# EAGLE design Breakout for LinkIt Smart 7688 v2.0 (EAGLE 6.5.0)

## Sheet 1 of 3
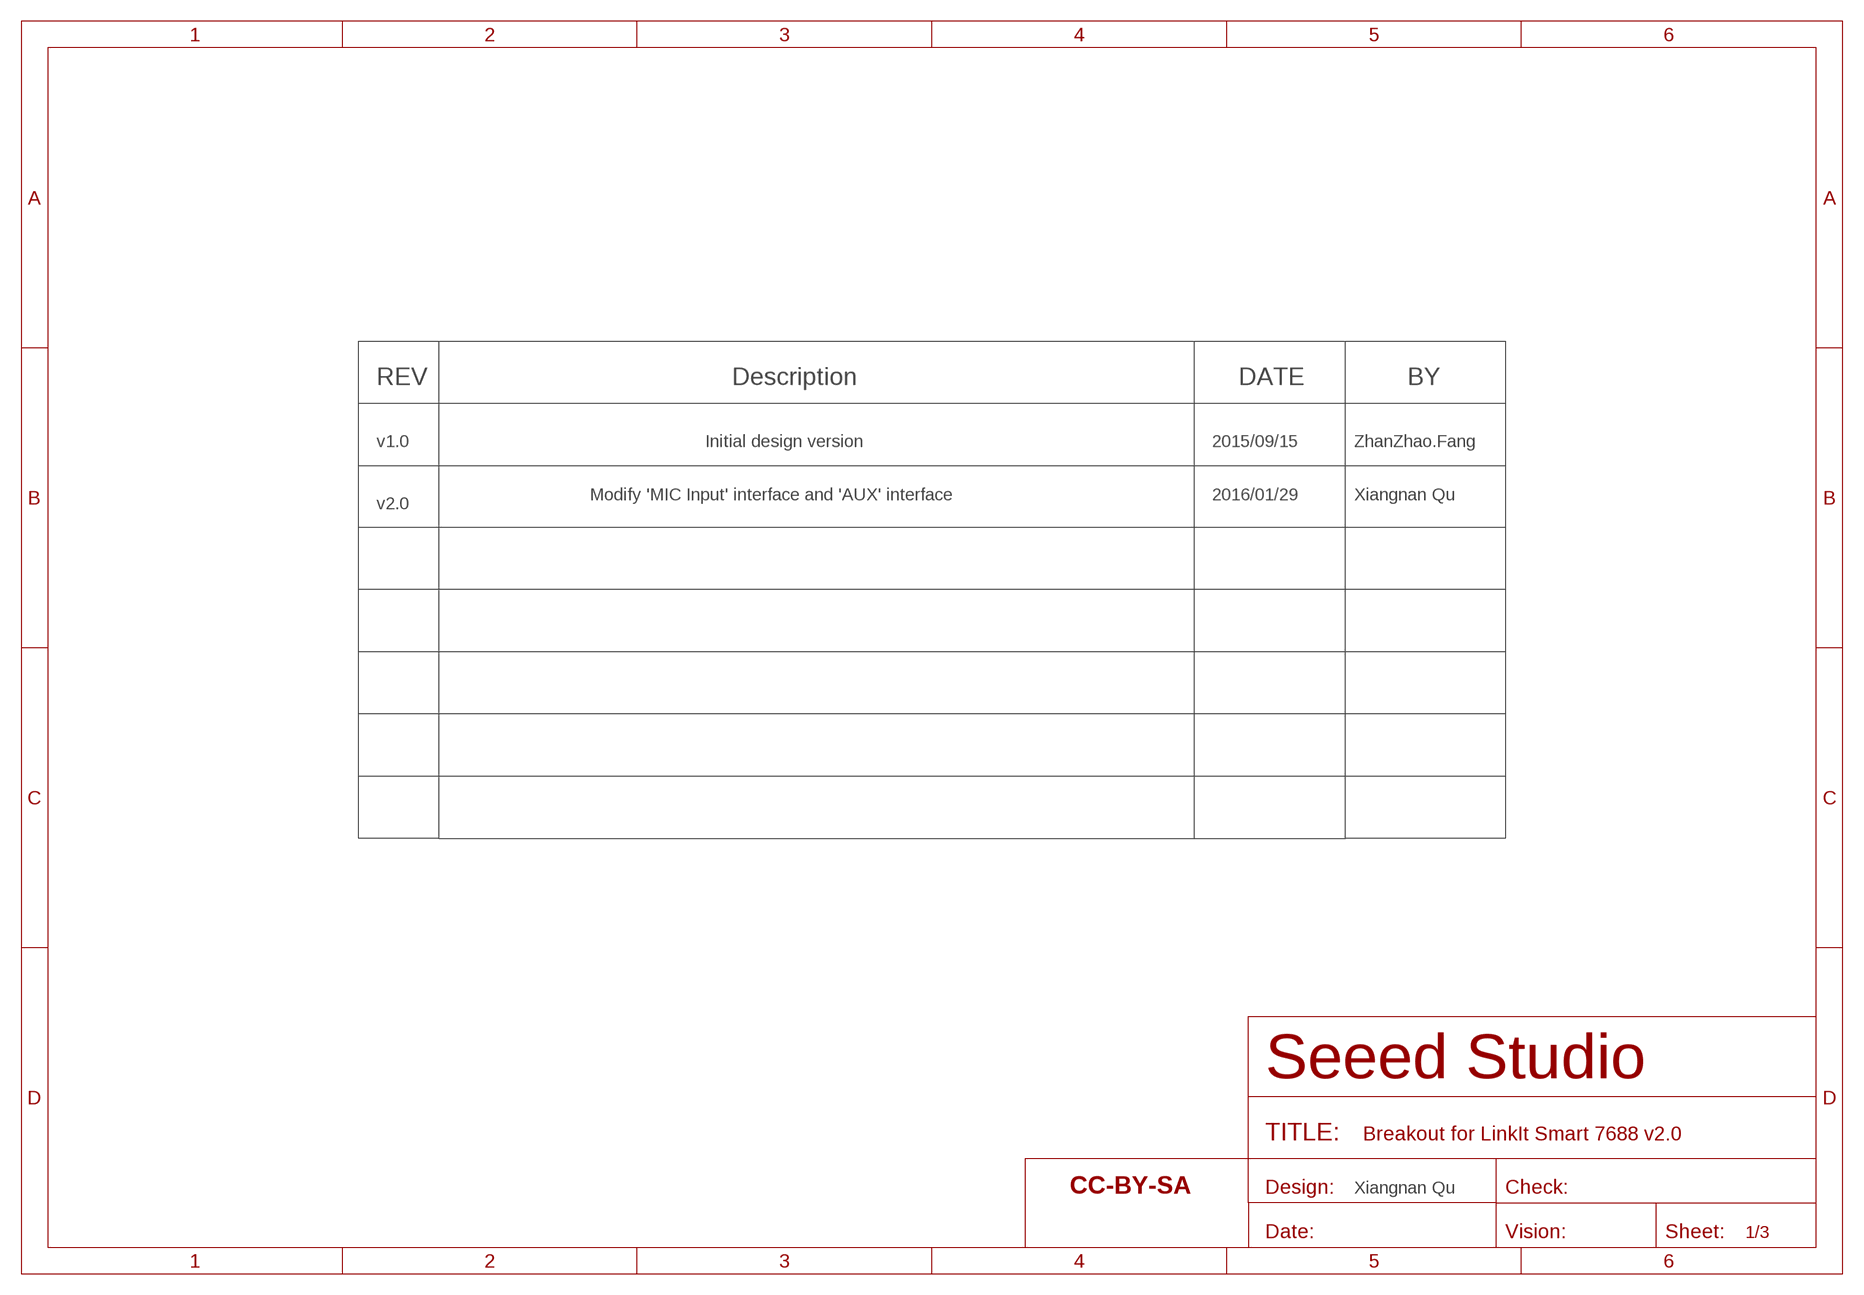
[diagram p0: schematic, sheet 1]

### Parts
FR2  DNP  SEEEDSTUDIO-OPEN-SCH-FRAME  [SEEEDSTUDIO-PCB-FRAME]

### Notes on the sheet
- REV | Description | DATE | BY
- v1.0 | Initial design version | 2015/09/15 | ZhanZhao.Fang
- Modify 'MIC Input' interface and 'AUX' interface | 2016/01/29 | Xiangnan Qu
- v2.0
- Xiangnan Qu

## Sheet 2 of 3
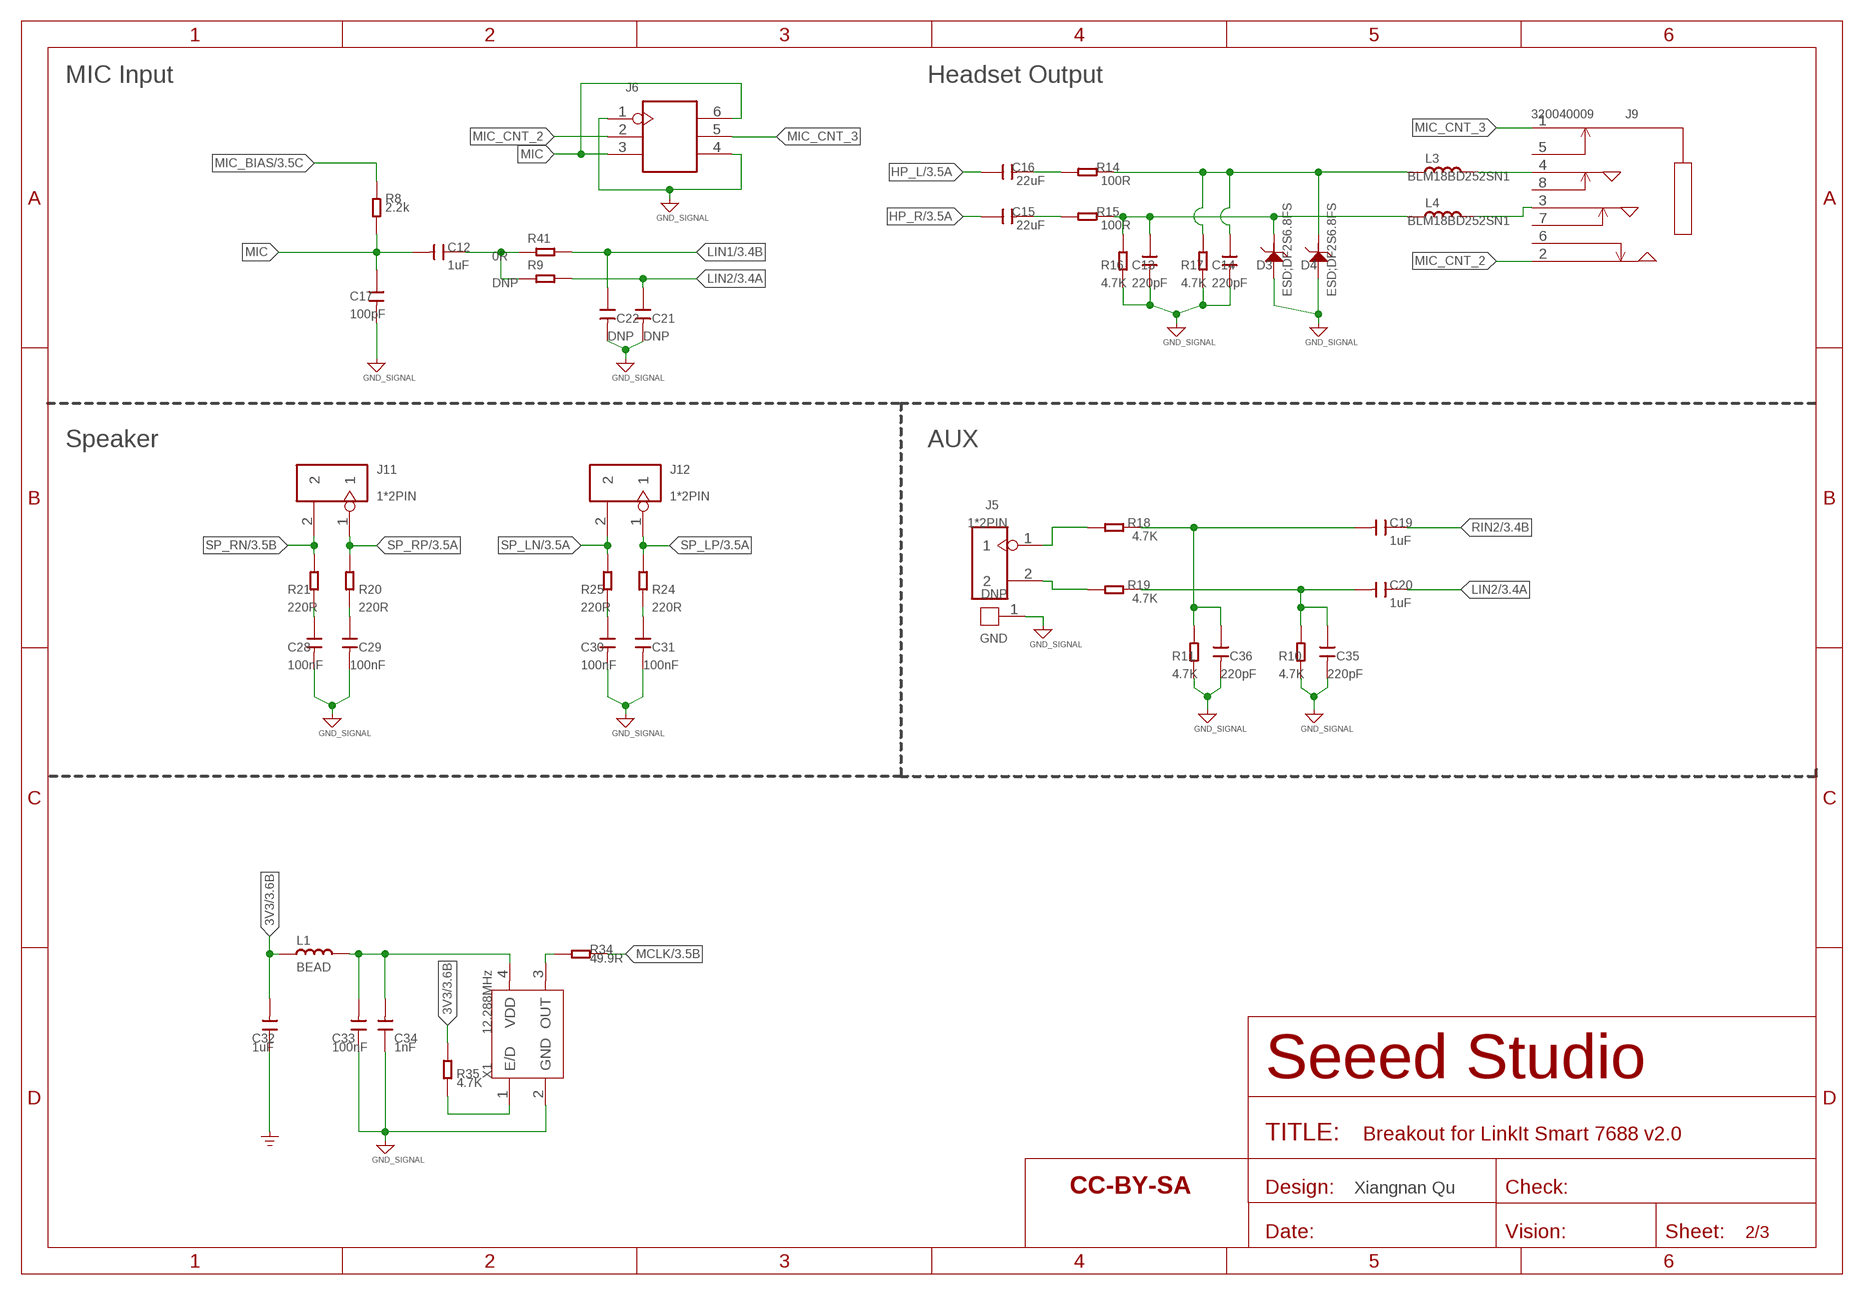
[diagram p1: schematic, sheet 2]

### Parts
C12  1uF  CAP-0603  [C0603]
C13  220pF  CAP-0603  [C0603]
C14  220pF  CAP-0603  [C0603]
C15  22uF  CAP-0805  [C0805]
C16  22uF  CAP-0805  [C0805]
C17  100pF  CAP-0603  [C0603]
C19  1uF  CAP-0603  [C0603]
C20  1uF  CAP-0603  [C0603]
C21  DNP  CAP-0603  [C0603]
C22  DNP  CAP-0603  [C0603]
C28  100nF  CAP-0603  [C0603]
C29  100nF  CAP-0603  [C0603]
C30  100nF  CAP-0603  [C0603]
C31  100nF  CAP-0603  [C0603]
C32  1uF  CAP-0805  [C0805]
C33  100nF  CAP-0603  [C0603]
C34  1nF  CAP-0603  [C0603]
C35  220pF  CAP-0603  [C0603]
C36  220pF  CAP-0603  [C0603]
D3  ESD;DF2S6.8FS  D-ESD-2P'DF2S6.8FS'  [SOD-923]
D4  ESD;DF2S6.8FS  D-ESD-2P'DF2S6.8FS'  [SOD-923]
FR3  DNP  SEEEDSTUDIO-OPEN-SCH-FRAME  [SEEEDSTUDIO-PCB-FRAME]
GND  DNP  HEADER-1P-40  [1P-80/40MIL]
J5  1*2PIN  HEADER-2P-65/35MIL  [H2-2.54]
J6  HEADER-2X3P'2.0'  [H2X3-2.0]
J9  320040009  AUDIO-JACK-8P-SMD'PJ-393'  [AUDIO8P-SMD-3.5-14.5X6.1X4.0MM]
J11  1*2PIN  HEADER-2P-65/35MIL  [H2-2.54]
J12  1*2PIN  HEADER-2P-65/35MIL  [H2-2.54]
L1  BEAD  INDUCTOR/FERRITE-BEAD'0603'  [L0603]
L3  BLM18BD252SN1  INDUCTOR/FERRITE-BEAD'0603'  [L0603]
L4  BLM18BD252SN1  INDUCTOR/FERRITE-BEAD'0603'  [L0603]
R8  2.2k  RES-0603  [R0603]
R9  DNP  RES-0603  [R0603]
R10  4.7K  RES-0603  [R0603]
R11  4.7K  RES-0603  [R0603]
R14  100R  RES-0603  [R0603]
R15  100R  RES-0603  [R0603]
R16  4.7K  RES-0603  [R0603]
R17  4.7K  RES-0603  [R0603]
R18  4.7K  RES-0603  [R0603]
R19  4.7K  RES-0603  [R0603]
R20  220R  RES-0603  [R0603]
R21  220R  RES-0603  [R0603]
R24  220R  RES-0603  [R0603]
R25  220R  RES-0603  [R0603]
R34  49.9R  RES-0603  [R0603]
R35  4.7K  RES-0603  [R0603]
R41  0R  RES-0603  [R0603]
X1  12.288MHz  CRYSTAL-4P(FXO-HC53)  [X4-SMD-5.15X3.35X1.4MM]

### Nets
3V3: C32.2 L1.1 R35.1 ; also sheet 3
AGND: C13.2 C14.2 C17.2 C21.2 C22.2 C28.2 C29.2 C30.2 C31.2 C33.1 C34.1 C35.2 C36.2 D3.2 D4.2 GND.1 J6.1 J6.4 R10.2 R11.2 R16.2 R17.2 X1.2(GND) ; supply symbol labelled GND_SIGNAL ; also sheet 3
GND: C32.1 ; supply symbol labelled GND_POWER ; also sheet 3
HP_L: C16.1 ; also sheet 3
HP_R: C15.1 ; also sheet 3
LIN1: C22.1 R41.2 ; also sheet 3
LIN2: C20.1 C21.1 R9.2 ; also sheet 3
MCLK: R34.1 ; also sheet 3
MIC: C12.2 C17.1 J6.3 J6.6 R8.1
MIC_BIAS: R8.2 ; also sheet 3
MIC_CNT_2: J6.2 J9.2
MIC_CNT_3: J6.5 J9.1
N$2: C12.1 R9.1 R41.1
N$7: C13.1 D3.1 L4.1 R15.1 R16.1
N$9: C19.2 C36.1 R11.1 R18.2
N$11: C20.2 C35.1 R10.1 R19.2
N$15: C28.1 R21.2
N$16: C29.1 R20.2
N$20: R34.2 X1.3(OUT)
N$25: C33.2 C34.2 L1.2 X1.4(VDD)
N$26: C30.1 R25.2
N$27: C31.1 R24.2
N$28: R35.2 X1.1(E/D)
N$29: J9.4 L3.2
N$30: J9.3 L4.2
N$31: C14.1 D4.1 L3.1 R14.1 R17.1
N$32: C16.2 R14.2
N$33: C15.2 R15.2
N$35: J5.1 R18.1
N$36: J5.2 R19.1
RIN2: C19.1 ; also sheet 3
SP_LN: J12.2 R25.1 ; also sheet 3
SP_LP: J12.1 R24.1 ; also sheet 3
SP_RN: J11.2 R21.1 ; also sheet 3
SP_RP: J11.1 R20.1 ; also sheet 3
Unconnected: J9.5 J9.6 J9.7 J9.8

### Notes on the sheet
- MIC Input | Headset Output
- Speaker | AUX
- Xiangnan Qu

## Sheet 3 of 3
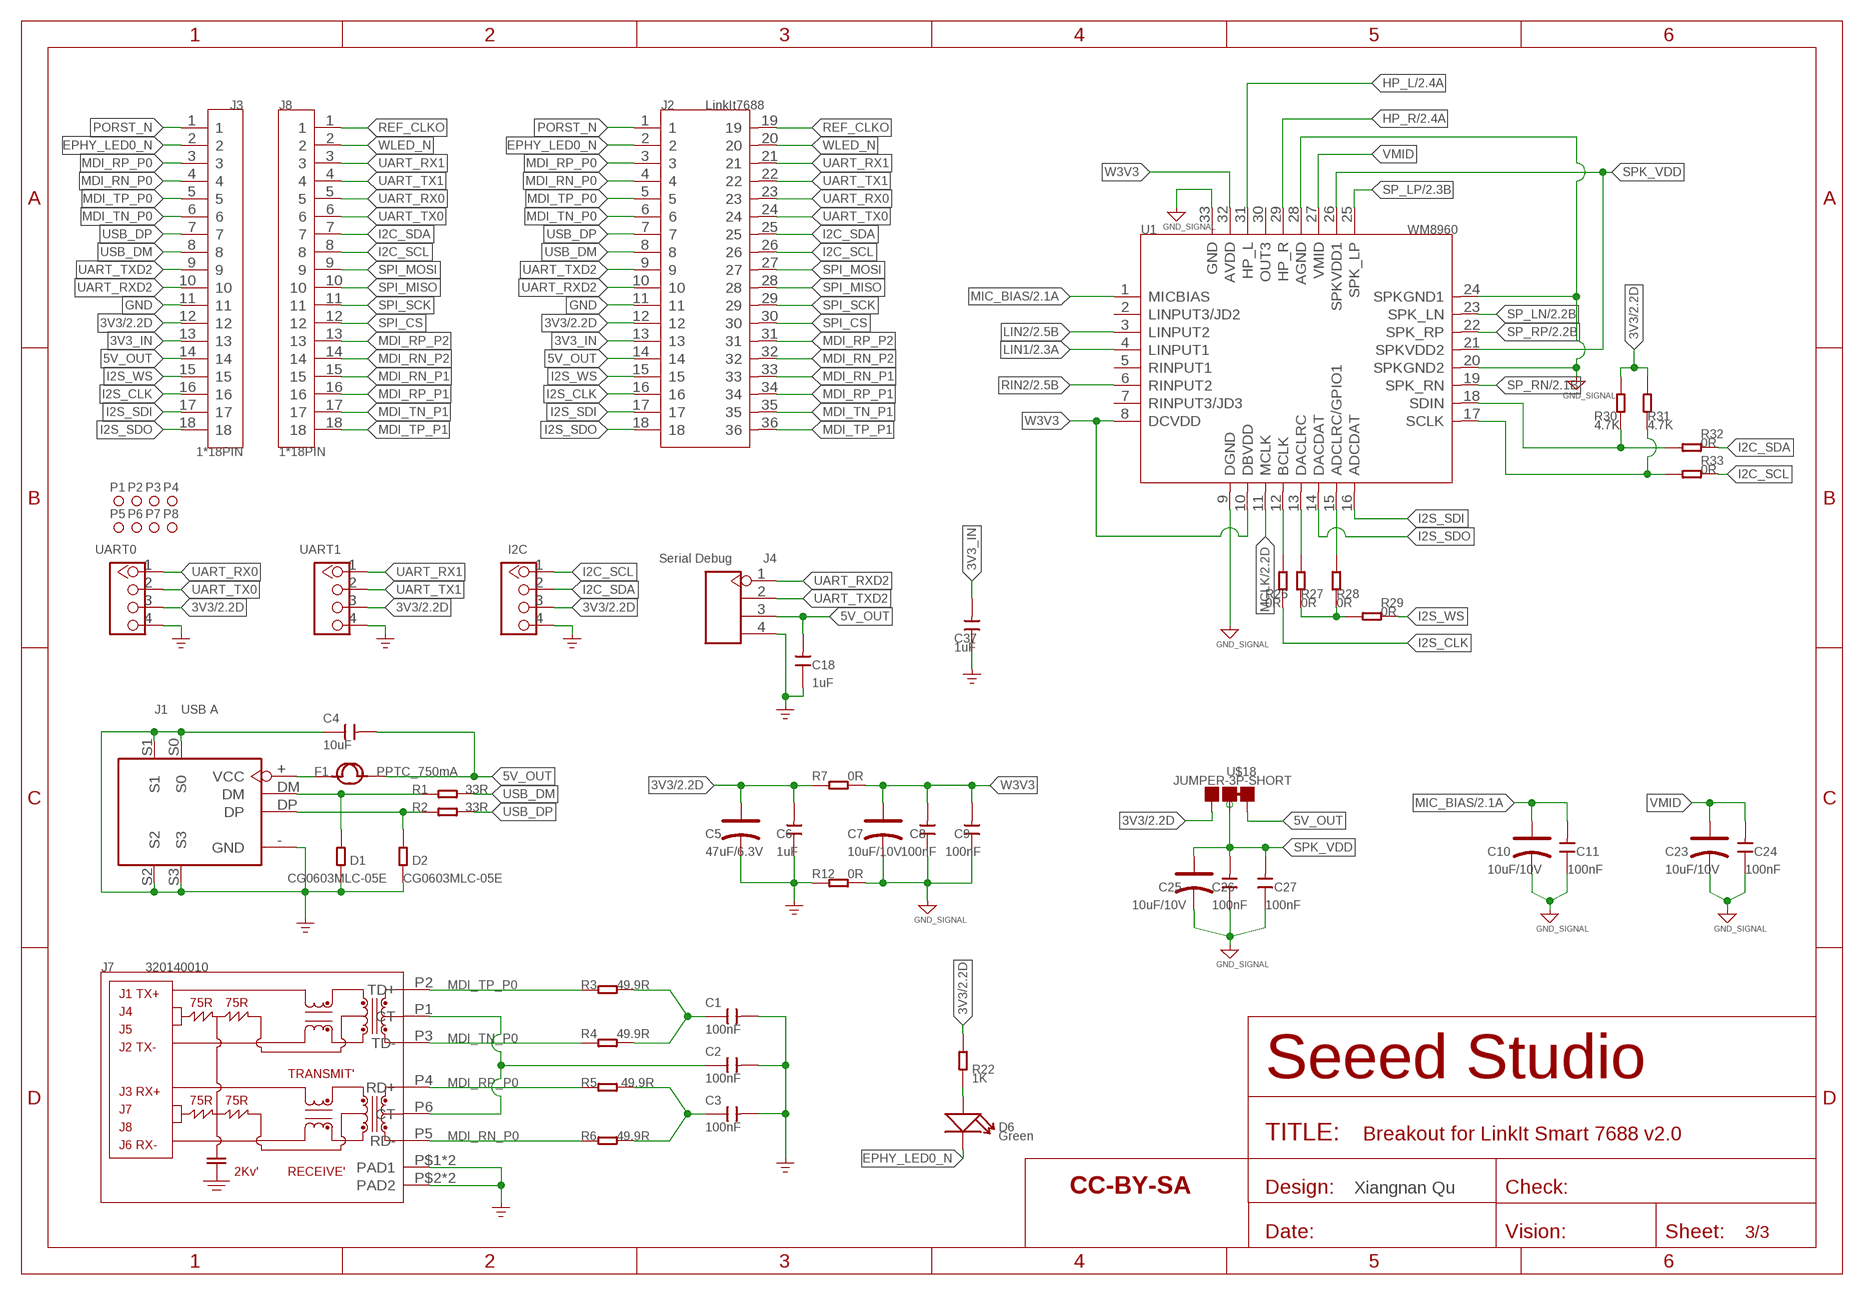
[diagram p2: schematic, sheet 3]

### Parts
C1  100nF  CAP-0603  [C0603]
C2  100nF  CAP-0603  [C0603]
C3  100nF  CAP-0603  [C0603]
C4  10uF  CAP-0805  [C0805]
C5  47uF/6.3V  CAP-POLAR-AVX-A  [AVX-A]
C6  1uF  CAP-0603  [C0603]
C7  10uF/10V  CAP-POLAR-AVX-A  [AVX-A]
C8  100nF  CAP-0603  [C0603]
C9  100nF  CAP-0603  [C0603]
C10  10uF/10V  CAP-POLAR-AVX-A  [AVX-A]
C11  100nF  CAP-0603  [C0603]
C18  1uF  CAP-0603  [C0603]
C23  10uF/10V  CAP-POLAR-AVX-A  [AVX-A]
C24  100nF  CAP-0603  [C0603]
C25  10uF/10V  CAP-POLAR-AVX-A  [AVX-A]
C26  100nF  CAP-0603  [C0603]
C27  100nF  CAP-0603  [C0603]
C37  1uF  CAP-0603  [C0603]
D1  CG0603MLC-05E  RES-0603  [R0603]
D2  CG0603MLC-05E  RES-0603  [R0603]
D6  Green  LED'0603'  [LED-0603]
F1  PPTC_750mA  FUSE'1206'  [F1206]
FR1  DNP  SEEEDSTUDIO-OPEN-SCH-FRAME  [SEEEDSTUDIO-PCB-FRAME]
I2C  320110033  GROVE-CONNECTOR-DIP-2.0  [HW4-2.0]
J1  USB A  USB4+4P-13.2X14.5  [USB4+4-90D-IN]
J2  LinkIt7688  LINKIT-7688  [HEADER-2X18P-2.54-65/35MIL]
J3  1*18PIN  HEADER-18P  [H18-2.54]
J4  Serial Debug  HEADER-4P-65/35MIL  [H4-2.54]
J7  320140010  RJ45-MJ6-BX11-RVS1T073  [RJ45-MJ6-BX11-RVS1T073]
J8  1*18PIN  HEADER-18P  [H18-2.54]
P1  NC  MARK-1.0'ANNULAR'  [ROUND-MARK-1.0]
P2  NC  MARK-1.0'ANNULAR'  [ROUND-MARK-1.0]
P3  NC  MARK-1.0'ANNULAR'  [ROUND-MARK-1.0]
P4  NC  MARK-1.0'ANNULAR'  [ROUND-MARK-1.0]
P5  NC  MARK-1.0'ANNULAR'  [ROUND-MARK-1.0]
P6  NC  MARK-1.0'ANNULAR'  [ROUND-MARK-1.0]
P7  NC  MARK-1.0'ANNULAR'  [ROUND-MARK-1.0]
P8  NC  MARK-1.0'ANNULAR'  [ROUND-MARK-1.0]
R1  33R  RES-0603  [R0603]
R2  33R  RES-0603  [R0603]
R3  49.9R  RES-0603  [R0603]
R4  49.9R  RES-0603  [R0603]
R5  49.9R  RES-0603  [R0603]
R6  49.9R  RES-0603  [R0603]
R7  0R  RES-0603  [R0603]
R12  0R  RES-0603  [R0603]
R22  1K  RES-0603  [R0603]
R26  0R  RES-0603  [R0603]
R27  0R  RES-0603  [R0603]
R28  0R  RES-0603  [R0603]
R29  0R  RES-0603  [R0603]
R30  4.7K  RES-0603  [R0603]
R31  4.7K  RES-0603  [R0603]
R32  0R  RES-0603  [R0603]
R33  0R  RES-0603  [R0603]
U1  WM8960  AMPLIFIER-WM8960  [QFN32G-0.5-5X5MM]
U$18  JUMPER-3P-SHORT  [3P-SMD-SHORT]
UART0  320110033  GROVE-CONNECTOR-DIP-2.0  [HW4-2.0]
UART1  320110033  GROVE-CONNECTOR-DIP-2.0  [HW4-2.0]

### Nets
3V3: C5.+ C6.2 I2C.3 J2.12 J3.12 R7.1 R22.2 R30.1 R31.1 U$18.00(R) UART0.3 UART1.3 ; also sheet 2
3V3_IN: C37.2 J2.13 J3.13
5V_OUT: C4.2 C18.2 F1.2 J2.14 J3.14 J4.3 U$18.11(L)
AGND: C7.- C8.1 C9.1 C10.- C11.1 C23.- C24.1 C25.- C26.1 C27.1 R12.2 U1.9(DGND) U1.20(SPKGND2) U1.24(SPKGND1) U1.28(AGND) U1.33(GND) ; supply symbol labelled GND_SIGNAL ; also sheet 2
EPHY_LED0_N: D6.- J2.2 J3.2
GND: C1.2 C2.2 C3.2 C4.1 C5.- C6.1 C18.1 C37.1 D1.1 D2.1 I2C.4 J1.-(GND) J1.S0 J1.S1 J1.S2 J1.S3 J2.11 J3.11 J4.4 J7.P$1(PAD1) J7.P$2(PAD2) J7.PAD1 J7.PAD2 R12.1 UART0.4 UART1.4 ; supply symbol labelled GND_POWER ; also sheet 2
HP_L: U1.31(HP_L) ; also sheet 2
HP_R: U1.29(HP_R) ; also sheet 2
I2C_SCL: I2C.1 J2.26 J8.8 R33.2
I2C_SDA: I2C.2 J2.25 J8.7 R32.2
I2S_CLK: J2.16 J3.16 R26.2
I2S_SDI: J2.17 J3.17 U1.16(ADCDAT)
I2S_SDO: J2.18 J3.18 U1.14(DACDAT)
I2S_WS: J2.15 J3.15 R29.2
LIN1: U1.4(LINPUT1) ; also sheet 2
LIN2: U1.3(LINPUT2) ; also sheet 2
MCLK: U1.11(MCLK) ; also sheet 2
MDI_RN_P0: J2.4 J3.4 J7.P5(RD-) R6.1
MDI_RN_P1: J2.33 J8.15
MDI_RN_P2: J2.32 J8.14
MDI_RP_P0: J2.3 J3.3 J7.P4(RD+) R5.1
MDI_RP_P1: J2.34 J8.16
MDI_RP_P2: J2.31 J8.13
MDI_TN_P0: J2.6 J3.6 J7.P3(TD-) R4.1
MDI_TN_P1: J2.35 J8.17
MDI_TP_P0: J2.5 J3.5 J7.P2(TD+) R3.1
MDI_TP_P1: J2.36 J8.18
MIC_BIAS: C10.+ C11.2 U1.1(MICBIAS) ; also sheet 2
N$1: D6.+ R22.1
N$3: D2.2 J1.DP R2.1
N$4: D1.2 J1.DM R1.1
N$5: F1.1 J1.+(VCC)
N$6: C2.1 J7.P1(CT) J7.P6(CT)
N$10: C1.1 R3.2 R4.2
N$12: C3.1 R5.2 R6.2
N$18: R26.1 U1.12(BCLK)
N$19: R27.1 U1.13(DACLRC)
N$21: R28.1 U1.15(ADCLRC/GPIO1)
N$22: R27.2 R28.2 R29.1
N$23: R31.2 R33.1 U1.17(SCLK)
N$24: R30.2 R32.1 U1.18(SDIN)
PORST_N: J2.1 J3.1
REF_CLKO: J2.19 J8.1
RIN2: U1.6(RINPUT2) ; also sheet 2
SP_LN: U1.23(SPK_LN) ; also sheet 2
SP_LP: U1.25(SPK_LP) ; also sheet 2
SP_RN: U1.19(SPK_RN) ; also sheet 2
SP_RP: U1.22(SPK_RP) ; also sheet 2
SPI_CS: J2.30 J8.12
SPI_MISO: J2.28 J8.10
SPI_MOSI: J2.27 J8.9
SPI_SCK: J2.29 J8.11
SPK_VDD: C25.+ C26.2 C27.2 U1.21(SPKVDD2) U1.26(SPKVDD1) U$18.MM(C)
UART_RX0: J2.23 J8.5 UART0.1
UART_RX1: J2.21 J8.3 UART1.1
UART_RXD2: J2.10 J3.10 J4.1
UART_TX0: J2.24 J8.6 UART0.2
UART_TX1: J2.22 J8.4 UART1.2
UART_TXD2: J2.9 J3.9 J4.2
USB_DM: J2.8 J3.8 R1.2
USB_DP: J2.7 J3.7 R2.2
VMID: C23.+ C24.2 U1.27(VMID)
W3V3: C7.+ C8.2 C9.2 R7.2 U1.8(DCVDD) U1.10(DBVDD) U1.32(AVDD)
WLED_N: J2.20 J8.2
Unconnected: U1.2(LINPUT3/JD2) U1.5(RINPUT1) U1.7(RINPUT3/JD3) U1.30(OUT3)

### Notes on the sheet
- Xiangnan Qu

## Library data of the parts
C1-C4 C6 C8 C9 C11-C22 C24 C26-C37 = Discrete-new:CAP: Ceramic Capacitors
C5 C7 C10 C23 C25 = Discrete-new:CAP-POLAR: Electrolytic Capacitors,Tantalum Capacitors and Super Capacitors
D1 D2 R1-R12 R14-R22 R24-R35 R41 = Discrete-new:RES
D3 D4 = Discrete-new:D-ESD-2P: SOD-923:304060009;SOD-123:304060001
D6 = Discrete-new:LED
F1 = Discrete-new:FUSE
FR1-FR3 = moudle-new:SEEEDSTUDIO-OPEN-SCH-FRAME
GND = Connector-new:HEADER-1P
I2C UART0 UART1 = Connector-new:GROVE-CONNECTOR-DIP: 4P-2.0:320110033;4P-2.0-90D:320110034
J1 = Connector-new:USB4+4P: 320010017 USB-A-FEMALE
J2 = template:LINKIT-7688
J3 J8 = Connector-new:HEADER-18P
J4 = Connector-new:HEADER-4P
J5 J11 J12 = Connector-new:HEADER-2P
J6 = Connector-new:HEADER-2X3P
J7 = Connector-new:RJ45-MJ6-BX11-RVS1T073: 320140010
J9 = Connector-new:AUDIO-JACK-8P-SMD: 320040009
L1 L3 L4 = Discrete-new:INDUCTOR/FERRITE-BEAD
P1-P8 = Discrete-new:MARK-1.0; PARTNO: DNP
U1 = template:AMPLIFIER-WM8960
U$18 = Discrete-new:JUMPER-3P-SHORT
X1 = template:CRYSTAL-4P(FXO-HC53)

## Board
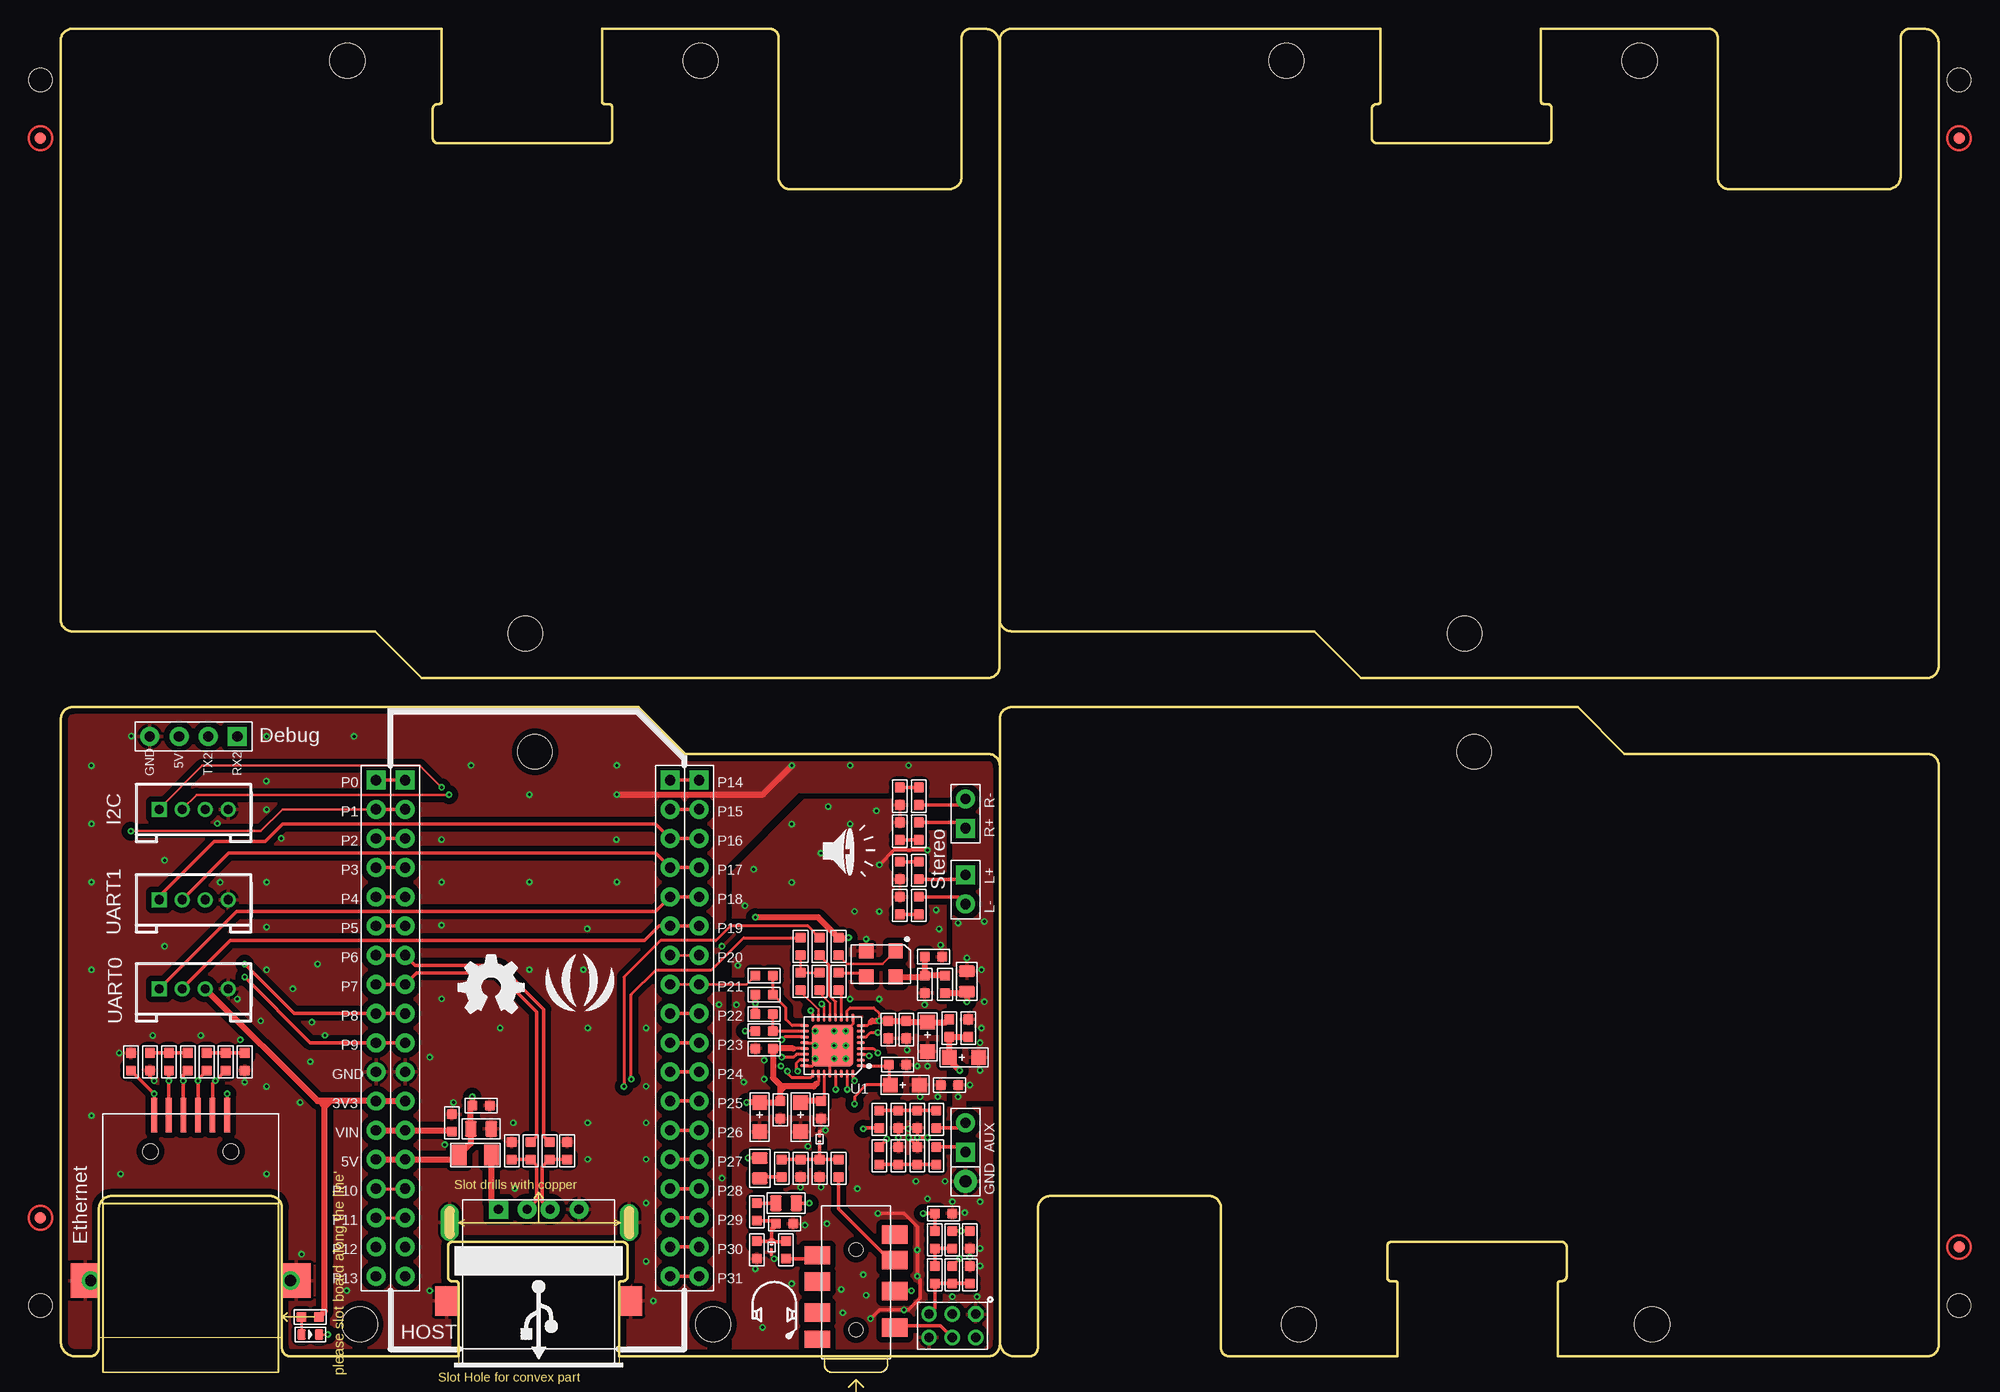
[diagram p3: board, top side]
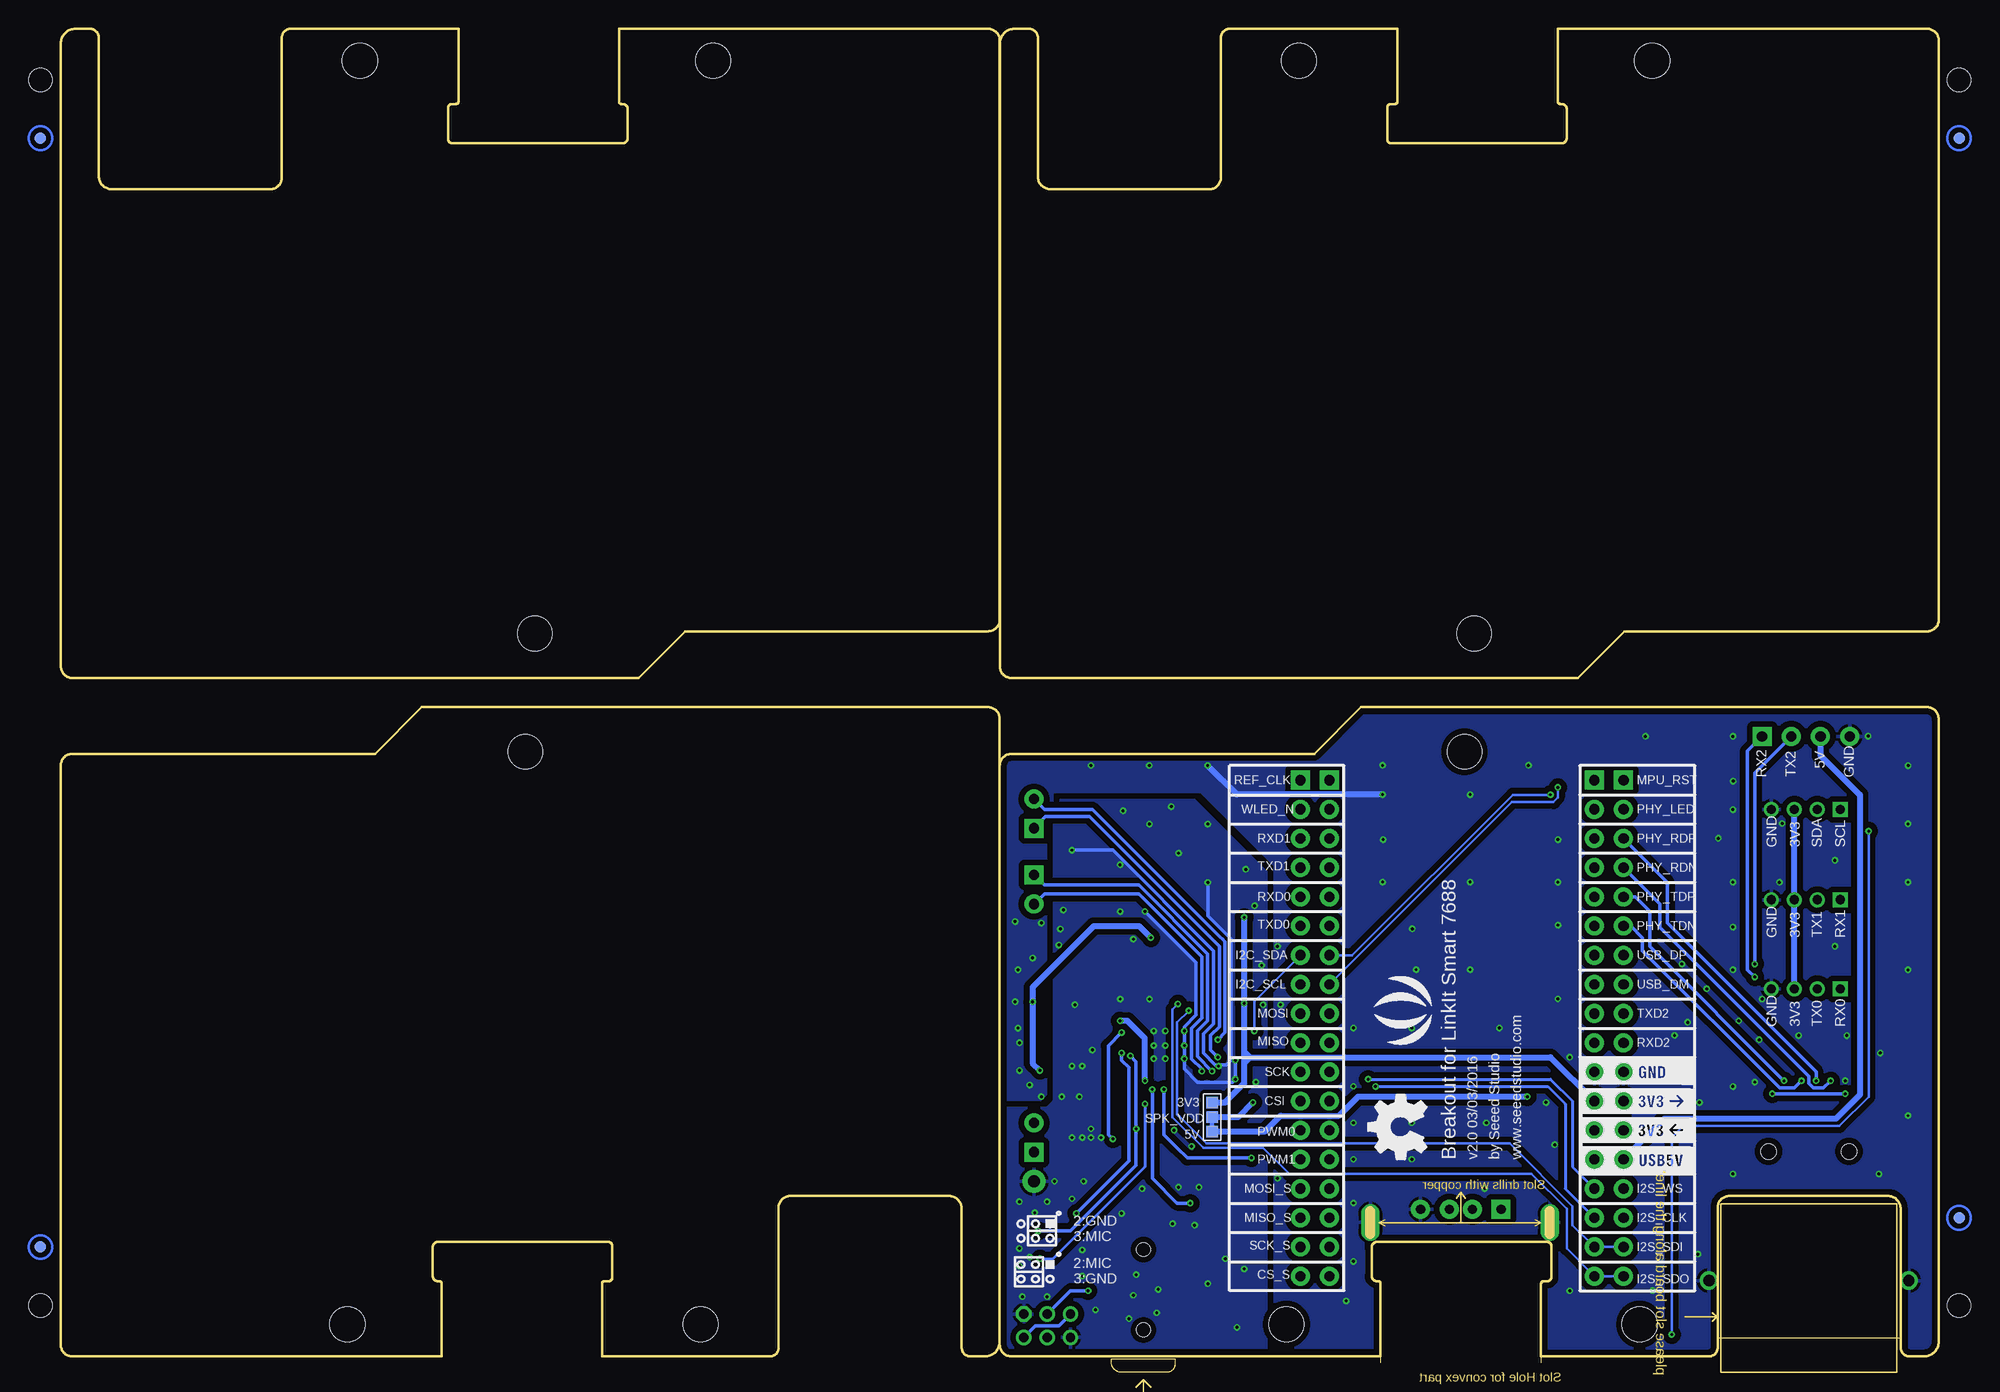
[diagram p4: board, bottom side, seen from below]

Size 163.47 x 116.15 mm. Coordinates in mm from the lower left corner, seen from the top.
Outline: 128 segments
Copper layers (1*16): Top 0.035mm / dielectric 1.5mm / Bottom 0.035mm
Design rules "SeeedStudio_2layer_DRU_no_angle_20140221 *": minimum track width 1mil, minimum drill 10mil, track to track 6mil, track to pad 6mil, pad to pad 6mil, via to via 6mil, smd to smd 0mil, copper to edge 10mil, drill to drill 10mil, minimum pad ring 10mil, minimum via ring 6mil, stop-mask expansion 2mil, vias tented up to drill 25mil, thermal gap 10mil
Holes 3 mm at 41.28,53.21 123.02,53.21 122.18,63.5 40.45,63.5
Holes 3.05 mm at 26.04,3.37 56.78,3.37 107.78,3.37 138.51,3.37 137.42,113.35 106.69,113.35 55.69,113.35 24.96,113.35
Holes 2.03 mm at -1.77,5.02 -1.77,111.7 165.24,111.7 165.24,5.02

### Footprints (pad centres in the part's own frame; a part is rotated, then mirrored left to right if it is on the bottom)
C0603 = smd 0.889 x 0.889: 1 0,0.762; 2 0,-0.762
C0805 = smd 1.397 x 1.016: 1 0,0.889; 2 0,-0.889
AVX-A = smd 1.27 x 1.27: + -1.27,0; - 1.27,0
R0603 = smd 0.889 x 0.889: 1 0,0.762; 2 0,-0.762
SOD-923 = smd 0.7 x 0.3: 1 -0.45,0; 2 0.45,0
LED-0603 = smd 0.762 x 0.889: + -0.762,0; - 0.762,0
F1206 = smd 1.27 x 1.778: 1 -1.397,0; 2 1.397,0
1P-80/40MIL = drill 1.016 pad 2.032: 1 0,0
HW4-2.0 = drill 0.8 pad 1.27 square: 1 -3,0 | drill 0.8 pad 1.27: 2 -1,0; 3 1,0; 4 3,0
USB4+4-90D-IN = drill 0.813 pad 1.651 square: + 0.85,-3.5 | drill 0.813 pad 1.651: - 0.85,3.5; DM 0.85,-1; DP 0.85,1 | smd 2.54 x 2.032: S0 8.83,8.001; S3 8.83,-8.001 | drill 0.7 pad 1.6 long: S1 2,7.874; S2 2,-7.747
HEADER-2X18P-2.54-65/35MIL = drill 0.889 pad 1.651 square: 1 0,21.59; 19 23.05,21.59 | drill 0.889 pad 1.651: 2 0,19.05; 3 0,16.51; 4 0,13.97; 5 0,11.43; 6 0,8.89; 7 0,6.35; 8 0,3.81; 9 0,1.27; 10 0,-1.27; 11 0,-3.81; 12 0,-6.35; 13 0,-8.89; 14 0,-11.43; 15 0,-13.97; 16 0,-16.51; 17 0,-19.05; 18 0,-21.59; 20 23.05,19.05; 21 23.05,16.51; 22 23.05,13.97; 23 23.05,11.43; 24 23.05,8.89; 25 23.05,6.35; 26 23.05,3.81; 27 23.05,1.27; 28 23.05,-1.27; 29 23.05,-3.81; 30 23.05,-6.35; 31 23.05,-8.89; 32 23.05,-11.43; 33 23.05,-13.97; 34 23.05,-16.51; 35 23.05,-19.05; 36 23.05,-21.59
H18-2.54 = drill 0.889 pad 1.651 square: 1 0,-21.59 | drill 0.889 pad 1.651: 2 0,-19.05; 3 0,-16.51; 4 0,-13.97; 5 0,-11.43; 6 0,-8.89; 7 0,-6.35; 8 0,-3.81; 9 0,-1.27; 10 0,1.27; 11 0,3.81; 12 0,6.35; 13 0,8.89; 14 0,11.43; 15 0,13.97; 16 0,16.51; 17 0,19.05; 18 0,21.59
H4-2.54 = drill 0.889 pad 1.651 square: 1 0,3.81 | drill 0.889 pad 1.651: 2 0,1.27; 3 0,-1.27; 4 0,-3.81
H2-2.54 = drill 0.889 pad 1.651 square: 1 0,1.27 | drill 0.889 pad 1.651: 2 0,-1.27
H2X3-2.0 = drill 0.813 pad 1.27 octagon: 1 -1.016,2.032 | drill 0.813 pad 1.27: 2 -1.016,0; 3 -1.016,-2.032; 4 1.016,-2.032; 5 1.016,0; 6 1.016,2.032
RJ45-MJ6-BX11-RVS1T073 = smd 0.5 x 3: P1 3.175,14.4; P2 1.905,14.4; P3 0.635,14.4; P4 -0.635,14.4; P5 -1.905,14.4; P6 -3.175,14.4 | smd 2.5 x 3: P$1 -9.2,0; P$2 9.2,0 | drill 1 pad 1.6: PAD1 -8.7,0; PAD2 8.7,0 | hole 1.35: -3.5,11.24; 3.5,11.24
AUDIO8P-SMD-3.5-14.5X6.1X4.0MM = smd 1.6 x 2.25: 1 3.9,-3.375; 2 7.1,-3.375; 3 9.8,-3.375; 4 10.2,3.375; 6 5.2,3.375; 7 7.9,3.375; 8 12,-3.375 | smd 1.5 x 2.25: 5 2.9,3.375 | hole 1.2: 3.7,0; 10.7,0
L0603 = smd 0.889 x 0.889: 1 -0.762,0; 2 0.762,0
ROUND-MARK-1.0 = smd 1.016 x 1.016: P$1 0,0
QFN32G-0.5-5X5MM = smd 0.7 x 0.25: 1 -2.45,1.75; 2 -2.45,1.25; 3 -2.45,0.75; 4 -2.45,0.25; 5 -2.45,-0.25; 6 -2.45,-0.75; 7 -2.45,-1.25; 8 -2.45,-1.75; 17 2.45,-1.75; 18 2.45,-1.25; 19 2.45,-0.75; 20 2.45,-0.25; 21 2.45,0.25; 22 2.45,0.75; 23 2.45,1.25; 24 2.45,1.75 | smd 0.25 x 0.7: 9 -1.75,-2.45; 10 -1.25,-2.45; 11 -0.75,-2.45; 12 -0.25,-2.45; 13 0.25,-2.45; 14 0.75,-2.45; 15 1.25,-2.45; 16 1.75,-2.45; 25 1.75,2.45; 26 1.25,2.45; 27 0.75,2.45; 28 0.25,2.45; 29 -0.25,2.45; 30 -0.75,2.45; 31 -1.25,2.45; 32 -1.75,2.45 | smd 3.6 x 3.6: 33 0,0
3P-SMD-SHORT = smd 1.016 x 1.016: 00 -1.27,0; 11 1.27,0; MM 0,0
X4-SMD-5.15X3.35X1.4MM = smd 1.24 x 1.3: 1 -1.27,-1.125; 2 1.27,-1.125; 3 1.27,1.125; 4 -1.27,1.125

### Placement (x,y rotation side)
C1  16.01,26.23 0 top
C2  6.1,26.23 180 top
C3  7.76,26.23 0 top
C4  36.58,20.38 270 top
C5  78.62,26.61 0 top
C6  79,29.15 0 top
C7  75.45,28.38 270 top
C8  73.61,29.02 180 top
C9  72.02,29.02 180 top
C10  73.48,24.19 0 top
C11  72.84,25.97 270 top
C12  76.08,7.68 0 top
C13  66.05,16.95 0 top
C14  60.59,9.84 0 top
C15  60.84,16.95 0 top
C16  63.13,13.91 270 top
C17  79.13,7.68 180 top
C18  36.58,22.42 270 top
C19  71.26,18.03 0 top
C20  71.26,21.21 180 top
C21  79.13,10.73 0 top
C22  76.84,13.02 90 top
C23  64.4,21.4 270 top
C24  66.18,22.03 180 top
C25  60.84,21.4 270 top
C26  62.62,22.03 180 top
C27  61.22,27.37 90 top
C28  73.03,49.34 0 top
C29  73.03,46.29 180 top
C30  73.03,39.81 180 top
C31  73.03,42.86 0 top
C32  78.88,33.21 0 top
C33  75.19,32.96 180 top
C34  75.95,35.37 270 top
C35  72.91,21.21 0 top
C36  74.56,18.03 180 top
C37  34.04,20.89 0 top
D1  39.25,18.48 0 top
D2  44.08,18.48 0 top
D3  66.05,19.49 90 top
D4  61.86,10.1 270 top
D6  21.73,2.48 0 top
F1  36.08,18.1 180 top
FR1  not placed on the board
FR2  not placed on the board
FR3  not placed on the board
GND  78.75,15.81 0 top
I2C  11.57,48.2 0 top
J1  41.6,14.22 270 top
J2  29.98,29.15 0 top
J3  27.44,29.15 180 top
J4  11.57,54.55 270 top
J5  78.75,19.62 180 top
J6  77.61,3.24 270 top
J7  11.31,7.18 0 top
J8  55.57,29.15 180 top
J9  69.22,-0.83 90 top
J11  78.75,47.82 180 top
J12  78.75,41.21 0 top
L1  76.97,32.96 90 top
L3  63.13,9.84 270 top
L4  67.7,16.95 270 top
P1  -1.77,106.62 0 top
P2  -1.77,106.62 0 bottom
P3  165.24,106.62 0 top
P4  165.24,106.62 0 bottom
P5  165.24,10.1 0 top
P6  165.24,10.1 0 bottom
P7  -1.77,12.64 0 top
P8  -1.77,12.64 0 bottom
R1  40.9,18.48 180 top
R2  42.55,18.48 180 top
R3  14.36,26.23 180 top
R4  12.71,26.23 180 top
R5  11.06,26.23 180 top
R6  9.41,26.23 180 top
R7  77.35,29.15 180 top
R8  77.61,7.68 180 top
R9  77.61,10.73 180 top
R10  74.56,21.21 0 top
R11  72.91,18.03 180 top
R12  77.35,24.19 270 top
R14  60.59,13.14 180 top
R15  62.75,16.95 0 top
R16  64.4,16.95 0 top
R17  63,12.13 90 top
R18  76.21,18.03 0 top
R19  76.21,21.21 180 top
R20  74.68,46.29 0 top
R21  74.68,49.34 180 top
R22  21.73,4 90 top
R24  74.68,42.86 180 top
R25  74.68,39.81 0 top
R26  66.05,36.26 180 top
R27  66.05,33.21 180 top
R28  64.4,33.21 180 top
R29  64.4,36.26 180 top
R30  61.22,30.35 90 top
R31  61.22,32.07 90 top
R32  61.22,28.89 270 top
R33  61.22,33.72 270 top
R34  67.7,33.21 180 top
R35  67.7,36.26 0 top
R41  76.08,10.73 180 top
U1  67.19,27.62 180 top
U$7  [OSHW_FILLX200_NOTEXT]  34.63,30.44 0 top
U$8  [SEEED-SILK-280*268MIL]  45.17,32.32 0 top
U$18  63.25,21.4 270 bottom
U$31  [OSHW_FILLX200_NOTEXT]  44.59,17.72 90 bottom
U$32  [SEEED-SILK-280*268MIL]  45.86,30.68 90 bottom
UART0  11.57,32.58 0 top
UART1  11.57,40.32 0 top
X1  71.38,34.73 180 top

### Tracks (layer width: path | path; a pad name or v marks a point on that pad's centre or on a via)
3V3  (via drill 0.25 pad 0.51)
  Top 0.508: R31.1 v60.46,31.31 R30.1 | v60.46,38.8 65.92,38.8 R35.1 v68.59,37.02 | C6.2 R7.1 C5.+ 77.35,26.35 v78.24,25.46 | L1.1 78.75,32.19 C32.2 v78.88,31.43 | J2.12 J3.12 23.5,22.8 | 23.5,22.8 23,22.8 | 23,22.8 22.49,22.8 | 22.49,22.8 22.34,22.8 UART0.3 | R22.2 23,4.51 23,22.29 | 23,22.29 23,22.8 | 23,22.29 22.49,22.8 | 23,22.29 23.5,22.8
  Bottom 0.508: v60.46,38.8 v60.46,31.31 60.46,27.11 | 60.46,26.61 59.95,26.61 | 59.95,26.61 33.79,26.61 J2.12 | 60.46,27.11 60.46,26.61 | 60.46,26.61 60.46,26.1 | 60.46,26.1 60.46,24.32 62.11,22.67 U$18.00 | 59.95,26.61 60.46,27.11 | 59.95,26.61 60.46,26.1 | UART0.3 UART1.3 I2C.3 | v78.24,25.46 78.88,26.1 v78.88,31.43 78.88,32.7 73.54,38.04 69.6,38.04 v68.59,37.02
3V3_IN
  Top 0.508: J3.13 J2.13 33.92,20.26 C37.2
5V_OUT  (via drill 0.25 pad 0.51)
  Top 0.508: v35.82,23.18 C18.2 35.7,22.29 C4.2 35.7,19.11 F1.2 34.3,17.72 J2.14 J3.14
  Bottom 0.508: J4.3 10.3,52.9 6.87,49.47 6.87,23.36 8.95,21.27 23.88,21.27 J3.14 | v35.82,23.18 50.55,23.18 52.21,21.53 57.29,21.53 58.68,20.13 U$18.11
AGND  (via drill 0.25 pad 0.51)
  Top 0.203: 65.92,26.35 65.79,26.35 v65.67,26.48 | 66.94,25.98 66.94,26.1 v67.32,26.48 | v67.32,27.62 67.07,27.87 66.18,27.87 66.18,28.38 v65.67,28.89
  Top 0.254: U1.28 66.94,25.98 | U1.24 65.44,25.87 65.92,26.35 67.06,26.35 | U1.20 66.18,27.87 | U1.9 68.94,29.5 v68.33,28.89
  Top 0.305: D3.2 66.05,20.13 66.18,20.26 v66.56,20.26 | v73.8,19.62 74.56,18.86 C36.2 v74.56,19.62 | v75.45,44.64 72.53,44.64 v71.26,43.37 | R11.2 v72.91,19.62 C35.2 73.73,20.45 v73.8,20.38 73.86,20.45 R10.2 v74.56,19.62 | v74.56,19.62 v75.45,19.62 | v70.48,3.86 71.26,4.64 73.8,4.64 74.81,5.65 74.81,7.3 v74.56,7.56 v74.56,9.84 74.56,11.87 73.41,13.02 v71.13,13.02
  Bottom 0.305: 61.35,26.35 v61.22,26.35 v61.22,24.7 61.48,24.45 64.52,24.45 65.67,25.59 65.67,29.27 64.65,30.29 64.65,34.86 v69.1,39.31 | 61.35,26.35 61.6,26.35 | 61.6,26.35 61.98,25.97 62.81,25.97 | v75.45,44.64 71.89,44.64 63.13,35.88 63.13,29.53 64.02,28.64 64.02,27.01 62.98,25.97 62.81,25.97 | 62.81,25.97 v62.68,25.84 | v63.62,41.83 63.62,38.91 61.6,36.89 61.6,26.61 | 61.6,26.61 61.6,26.35 | 61.6,26.61 61.35,26.35
  other vias: 75.19,31.18 73.67,27.24 76.59,36.39 70.11,36.89 71,48.07 68.33,27.62 67.32,28.89 68.33,26.48 65.03,18.86 60.46,8.19 64.78,12 64.4,15.3 66.18,15.3 76.97,15.81 80.02,14.03 66.16,44.37 63.62,46.91 71.24,39.29 71.24,31.67 68.7,31.67 63.62,6.91 67.94,6.4 61.08,3.1 68.7,46.91 59.44,24.45 58.81,31.18 58.94,34.61 59.56,39.8 74.56,25.84 75.45,25.84 74.81,23.18 76.34,23.18 65.67,27.62 74.43,15.81 77.61,14.03 78.69,13.08 80.02,9.97 69.35,15.18 79.76,5.78 77.61,5.78 79.13,9.21 80.02,8.45 66.68,12.13 69.86,7.68 75.45,14.29 73.4,4.62 68.07,4.37 70.1,5.89 60.32,42.98 66.8,48.44 76.2,39.42 76.45,37.77 62.1,9.07
  pour Top (isolate 0.508): 76.46,48.96 64.76,48.96 58.56,42.76 58.56,-0.7 82.05,-0.7 82.05,21.4 81.29,22.16 77.61,22.16 76.97,22.8 76.97,48.45
  pour Bottom (isolate 0.508): 76.46,48.96 64.78,48.96 58.56,42.73 58.56,-0.7 82.05,-0.7 82.05,21.4 81.29,22.16 77.61,22.16 76.97,22.8 76.97,48.45
EPHY_LED0_N  (via drill 0.25 pad 0.51)
  Top 0.203: J3.2 19.31,48.2 17.41,46.29 v6.1,46.29 | D6.- v23.25,2.48
  Top 0.305: J3.2 J2.2
  Bottom 0.203: v23.25,2.48 23.25,19.62 22.23,20.64 8.64,20.64 6.1,23.18 v6.1,46.29
GND  (via drill 0.25 pad 0.51)
  Top 0.305: C3.2 7.76,24.96 v8.14,24.57
  Top 0.508: v48.41,49.48 61.11,49.48 v63.64,52.01
  Bottom 0.508: v48.41,49.48 61.11,49.48 v63.64,52.01
  other vias: 79.13,24.19 78.11,23.18 5.09,26.99 16.01,24.45 15.38,31.69 8.01,28.51 80.15,29.15 80.15,34.23 78.87,35.25 73.79,52.01 68.71,52.01 6.14,54.57 13.63,46.97 13.87,41.85 2.67,52 2.67,46.93 2.67,41.85 2.67,34.23 5.21,16.45 17.91,16.45 17.91,24.07 17.91,34.23 17.91,41.85 17.91,54.55 25.53,54.55 33.15,41.85 33.15,31.69 32.12,26.61 32.12,6.29 50.95,8.84 50.95,13.92 50.95,24.08 50.95,29.16 45.87,29.16 40.79,34.24 40.79,41.86 48.41,41.86 40.79,49.48 35.71,52.02 48.41,52.02 45.49,34.24 38.25,29.16 2.67,21.53 17.9,50.65 17.91,48.18 19.19,45.67 17.91,37.95 33.15,38.11 33.15,45.57 48.36,45.55 45.83,37.8 51.58,5.41 57.55,16.08 57.55,36.27 57.3,31.19 21.85,29.66 22.99,28.52 39.52,15.19 33.42,19 34.18,22.68 39.39,20.9 45.87,20.9 50.95,20.9 50.95,17.73 45.87,17.73 9.04,43.76 9.04,36.27 12.2,28.51 20.2,32.58 22.36,34.73 15.63,28.13 17.41,29.78 20.96,9.47 24.9,6.29 20.84,22.68 21.72,26.23 78.11,38.29 80.4,38.42 80.4,31.44 80.02,27.88 80.02,25.47
  pour Bottom (isolate 0.508, rank 2): -0.5,57.72 82.05,57.72 82.05,-0.06 -0.5,-0.06
  pour Top (isolate 0.508, rank 2): -0.5,57.72 82.05,57.72 82.05,-0.06 -0.5,-0.06
HP_L  (via drill 0.25 pad 0.51)
  Top 0.254: U1.31 68.44,23.83 v68.46,23.81
  Top 0.305: C16.1 v65.16,13.91
  Bottom 0.305: v68.46,23.81 68.46,16.07 66.3,13.91 v65.16,13.91
HP_R  (via drill 0.25 pad 0.51)
  Top 0.254: U1.29 v67.44,23.82 v67.45,23.81
  Top 0.305: C15.1 v59.83,17.84
  Bottom 0.305: v67.45,23.81 67.45,19.88 66.43,18.86 66.3,18.73 65.41,17.84 v59.83,17.84
I2C_SCL  (via drill 0.25 pad 0.51)
  Top 0.203: R33.2 59.7,32.96 J8.8 J2.26 | I2C.1 8.57,48.24 12.33,52.01 31.25,52.01 v33.16,50.1
  Bottom 0.203: v33.16,50.1 33.16,49.21 33.54,48.83 37.16,48.83 J2.26
I2C_SDA  (via drill 0.25 pad 0.51)
  Top 0.203: R32.2 v59.57,28.89 | J8.7 J2.25 | I2C.2 10.57,48.21 11.82,49.47 v33.79,49.47
  Bottom 0.203: J8.7 59.57,31.5 v59.57,28.89 | v33.79,49.47 37.09,49.47 51.06,35.5 J2.25
I2S_CLK  (via drill 0.25 pad 0.51)
  Top 0.254: R26.2 65.03,38.04 58.3,38.04 57.03,36.77 52.21,36.77 49.03,33.59 v49.03,24.07 | J3.16 J2.16
  Bottom 0.254: v49.03,24.07 34.04,24.07 32.52,22.54 32.52,15.18 J2.16
I2S_SDI  (via drill 0.25 pad 0.51)
  Top 0.203: U1.16 65.44,30.52 v65.29,30.67
  Bottom 0.203: J3.17 J2.17 31.89,12 31.89,13.65 37.35,19.11 63.76,19.11 66.11,21.46 66.18,21.53 66.3,21.65 66.3,29.65 v65.29,30.67
I2S_SDO  (via drill 0.25 pad 0.51)
  Top 0.203: U1.14 66.44,31.04 v66.24,31.24
  Bottom 0.203: J3.18 J2.18 32.39,9.97 32.39,13.4 35.44,16.45 56.52,16.45 58.81,18.73 64.02,18.73 66.68,21.4 66.68,30.8 v66.24,31.24
I2S_WS  (via drill 0.25 pad 0.51)
  Top 0.254: v49.67,24.7 49.67,32.07 51.82,34.23 56.65,34.23 59.44,37.02 R29.2 | J3.15 J2.15
  Bottom 0.254: v49.67,24.7 33.79,24.7 31.89,22.8 31.89,17.08 J2.15
LIN1  (via drill 0.25 pad 0.51)
  Top 0.254: U1.4 70.74,27.37 v71.13,26.99
  Top 0.305: v75.07,13.02 C22.1 R41.2
  Bottom 0.305: v71.13,26.99 71.13,26.35 70.49,25.72 70.49,17.59 v75.07,13.02
LIN2  (via drill 0.25 pad 0.51)
  Top 0.254: U1.3 70.23,26.87 v70.37,26.73
  Top 0.305: C20.1 69.92,20.45 v69.86,20.38 | R9.2 v78.37,11.49 C21.1
  Bottom 0.305: v70.37,26.73 69.86,26.23 v69.86,20.38 69.86,17.21 75.57,11.49 v78.37,11.49
MCLK
  Top 0.254: U1.11 67.94,32.21 R34.1
MDI_RN_P0  (via drill 0.25 pad 0.51)
  Top 0.305: J7.P5 v9.41,24.57 R6.1 | J3.4 J2.4
  Bottom 0.305: v9.41,24.57 10.04,23.94 10.93,23.94 11.31,24.32 11.31,24.96 24.27,37.91 24.27,39.94 J3.4
MDI_RN_P1
  Top 0.305: J2.33 J8.15
MDI_RN_P2
  Top 0.305: J8.14 J2.32
MDI_RP_P0  (via drill 0.25 pad 0.51)
  Top 0.305: J7.P4 v10.68,24.57 10.68,25.08 R5.1 | J3.3 J2.3
  Bottom 0.305: v10.68,24.57 10.68,25.34 23.63,38.29 23.63,41.85 J3.3
MDI_RP_P1
  Top 0.305: J2.34 J8.16
MDI_RP_P2
  Top 0.305: J2.31 J8.13
MDI_TN_P0  (via drill 0.25 pad 0.51)
  Top 0.305: J7.P3 v11.95,24.57 11.95,24.7 R4.1 | J3.6 J2.6
  Bottom 0.305: v11.95,24.57 12.58,23.94 13.85,23.94 25.79,35.88 25.79,37.02 26.81,38.04 J3.6
MDI_TN_P1
  Top 0.305: J2.35 J8.17
MDI_TP_P0  (via drill 0.25 pad 0.51)
  Top 0.305: R3.1 v13.47,24.57 13.22,24.32 J7.P2 | J3.5 J2.5
  Bottom 0.305: J3.5 26.42,40.58 25.15,39.31 25.15,36.26 v13.47,24.57
MDI_TP_P1
  Top 0.305: J2.36 J8.18
MIC
  Top 0.305: C17.1 R8.1 C12.2 76.08,4.76 J6.3
  Bottom 0.305: J6.6 78.62,3.24 76.59,3.24 J6.3
MIC_BIAS  (via drill 0.25 pad 0.51)
  Top 0.254: U1.1 71.98,25.87 C11.2 72.08,24.32 C10.+ 70.11,24.19 69.1,23.18 v69.1,22.54 | R8.2 v78.24,9.08
  Bottom 0.254: v69.1,22.54 69.1,17.08 77.1,9.08 v78.24,9.08
MIC_CNT_2  (via drill 0.25 pad 0.51)
  Top 0.305: J9.2 74.04,6.27 v74.05,6.29
  Bottom 0.305: J6.2 75.57,6.29 v74.05,6.29
MIC_CNT_3
  Top 0.305: J6.5 76.59,3.24 72.76,3.24 J9.1
N$1
  Top 0.203: D6.+ R22.1
N$2
  Top 0.305: R9.1 R41.1 C12.1
N$3
  Top 0.305: J1.DP 42.58,13.37 41.92,14.03 41.92,17.08 R2.1 D2.2
N$4
  Top 0.305: J1.DM 40.62,13.37 41.41,14.16 41.41,17.21 R1.1 D1.2
N$5
  Top 0.508: F1.1 37.47,14 J1.+
N$6  (via drill 0.25 pad 0.51)
  Top 0.305: v14.49,23.43 J7.P1 | C2.1 v8.14,23.43 J7.P6
  Bottom 0.305: v8.14,23.43 v14.49,23.43
N$7
  Top 0.305: L4.1 C13.1 | C13.1 D3.1 | C13.1 R16.1 R15.1
N$9
  Top 0.305: R18.2 C36.1 R11.1 C19.2
N$10
  Top 0.305: C1.1 R3.2 R4.2
N$11
  Top 0.305: R19.2 R10.1 C35.1 C20.2
N$12
  Top 0.305: R5.2 R6.2 C3.1
N$15
  Top 0.305: C28.1 R21.2
N$16
  Top 0.305: C29.1 R20.2
N$18
  Top 0.254: U1.12 67.44,31.44 66.87,32 66.87,34.67 R26.1
N$19
  Top 0.203: U1.13 66.94,31.3 66.05,32.19 R27.1
N$20
  Top 0.254: R34.2 69.75,33.97 X1.3
N$21
  Top 0.203: U1.15 65.94,30.78 64.4,32.32 R28.1
N$22
  Top 0.203: R27.2 R28.2 R29.1
N$23
  Top 0.254: U1.17 63.66,29.37 63.13,29.91 63.13,30.92 R31.2 R33.1
N$24
  Top 0.254: U1.18 62,28.87 R32.1 R30.2
N$25
  Top 0.508: X1.4 75.08,33.61 C33.2 | C34.2 C33.2 | L1.2 C33.2
N$26
  Top 0.305: R25.2 C30.1
N$27
  Top 0.305: R24.2 C31.1
N$28
  Top 0.203: R35.2 68.46,34.73 71.53,34.73 X1.1
N$29
  Top 0.305: L3.2 65.55,9.08 J9.4
N$30
  Top 0.305: J9.3 72.12,8.97 67.7,13.4 L4.2
N$31
  Top 0.305: R14.1 61.98,12.38 R17.1 61.86,11.75 61.86,11.49 | 61.86,10.6 D4.1 62.05,10.55 | 61.86,10.6 61.86,10.86 | 61.86,10.86 61.86,11.24 61.86,11.49 | C14.1 61.6,10.6 | 61.67,10.6 61.86,10.6 | 61.6,10.6 61.86,10.86 | 61.6,10.6 61.67,10.6 | 61.67,10.6 61.86,10.41 | 62.17,10.55 63.07,10.55 L3.1 | 62.17,10.55 61.86,10.86 | 62.17,10.55 62.05,10.55 | 62.05,10.55 61.86,10.35 | 61.86,11.49 62.24,11.87
N$32
  Top 0.305: R14.2 C16.2
N$33
  Top 0.305: R15.2 60.97,16.19 C15.2
N$35
  Top 0.305: R18.1 78.3,18.8 J5.1
N$36
  Top 0.305: R19.1 78.3,20.45 J5.2
PORST_N
  Top 0.305: J3.1 J2.1
REF_CLKO
  Top 0.305: J2.19 J8.1
RIN2  (via drill 0.25 pad 0.51)
  Top 0.254: U1.6 70.1,28.37 70.49,28.77 v71.13,28.77
  Top 0.305: v71.89,19.49 71.89,19.43 C19.1
  Bottom 0.305: v71.13,28.77 72.27,27.62 72.27,19.88 v71.89,19.49
SP_LN  (via drill 0.25 pad 0.51)
  Top 0.254: U1.23 64.29,26.37 64.02,26.1 64.02,25.53 v64.14,25.4
  Top 0.305: R25.1 78.11,40.58 J12.2
  Bottom 0.305: J12.2 77.86,40.83 69.6,40.83 64.14,35.37 64.14,30.04 65.03,29.15 65.03,26.48 64.14,25.59 v64.14,25.4
SP_LP  (via drill 0.25 pad 0.51)
  Top 0.254: U1.25 65.44,24.98 65.29,24.83 63.64,24.83 63.25,25.21 v63.25,25.4
  Top 0.305: R24.1 78.37,42.1 J12.1
  Bottom 0.305: J12.1 77.86,41.59 69.6,41.59 63.64,35.62 63.64,29.78 64.52,28.89 64.52,26.67 v63.25,25.4
SP_RN  (via drill 0.25 pad 0.51)
  Top 0.254: U1.19 62.99,28.37 v62.75,28.13
  Top 0.305: R21.1 78.24,48.58 J11.2
  Bottom 0.305: J11.2 77.86,48.2 73.67,48.2 62.56,37.08 62.37,36.89 62.11,36.64 62.11,28.77 v62.75,28.13
SP_RP  (via drill 0.25 pad 0.51)
  Top 0.254: U1.22 64.03,26.87 63.76,26.61 v62.75,26.61
  Top 0.305: R20.1 78.24,47.05 J11.1
  Bottom 0.305: J11.1 77.73,47.56 73.92,47.56 63,36.64 62.87,36.51 62.62,36.26 62.62,29.27 63.38,28.51 63.38,27.24 v62.75,26.61
SPI_CS
  Top 0.305: J2.30 J8.12
SPI_MISO
  Top 0.305: J2.28 J8.10
SPI_MOSI
  Top 0.305: J2.27 J8.9
SPI_SCK
  Top 0.305: J2.29 J8.11
SPK_VDD  (via drill 0.25 pad 0.51)
  Top 0.254: U1.26 65.94,24.47 65.79,24.32 | U1.21 63.77,27.37 63.76,27.37
  Top 0.508: 63,24.07 65.54,24.07 65.79,24.32 | 63,24.07 62.62,24.07 | 62.62,24.07 62.62,24.19 61.98,24.83 C27.2 63.76,27.37 | 62.62,24.07 62.62,23.69 | 62.62,23.69 C26.2 62.49,22.67 C25.+ v59.7,22.67 | 63,24.07 62.62,23.69
  Bottom 0.508: v59.7,22.67 60.97,21.4 U$18.MM
UART_RX0
  Top 0.305: UART0.1 15.3,39.31 51.76,39.31 J2.23 J8.5
UART_RX1
  Top 0.305: UART1.1 8.64,40.32 8.64,40.7 13.34,45.4 17.79,45.4 19.31,46.93 51.76,46.93 J2.21 J8.3
UART_RXD2  (via drill 0.25 pad 0.51)
  Top 0.305: J2.10 J3.10 21.73,27.88 v16.01,33.59
  Bottom 0.305: J4.1 16.65,53.28 16.65,34.23 v16.01,33.59
UART_TX0
  Top 0.305: UART0.2 10.57,32.59 14.74,36.77 50.81,36.77 52.08,38.04 J2.24 J8.6
UART_TX1
  Top 0.305: UART1.2 14.63,44.39 51.76,44.39 J2.22 J8.4
UART_TXD2  (via drill 0.25 pad 0.51)
  Top 0.305: J2.9 J3.9 20.33,30.42 v16.01,34.73
  Bottom 0.305: v16.01,34.73 16.01,51.37 J4.2
USB_DM
  Top 0.305: R1.2 41.41,19.75 41.41,30.54 37.98,33.97 31,33.97 J2.8 J3.8
USB_DP
  Top 0.305: R2.2 42.05,19.75 42.05,30.8 38.24,34.61 30.87,34.61 J2.7 J3.7
VMID
  Top 0.254: U1.27 66.44,23.06 C24.2
  Top 0.508: C24.2 64.52,22.8 C23.+
W3V3  (via drill 0.25 pad 0.51)
  Top 0.254: U1.32 68.94,24.73 v69.1,24.57 | U1.8 70.21,29.37 70.49,29.65 | U1.10 68.44,30.65 68.72,30.92 70.75,30.92 71.26,30.42 71.26,30.16 71.26,30.04 | 71.26,30.04 v71.26,29.78 | 71.26,30.04 71.51,29.78 | 71.26,30.04 71,29.78
  Top 0.508: 70.49,29.65 70.62,29.78 71,29.78 v71.26,29.78 71.51,29.78 C9.2 C8.2 73.73,29.65 C7.+ 77.1,29.65 R7.2
  Bottom 0.508: v69.1,24.57 69.1,28.26 70.62,29.78 v71.26,29.78
WLED_N
  Top 0.305: J2.20 J8.2

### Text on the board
tPlace: Debug | 5V | GND | TX2 | RX2 | P0 | P14 | R- | I2C | P1 | P15 | R+ | P2 | P16 | P3 | P17 | L+ | Stereo | P4 | P18 | L- | UART1 | P5 | P19 | P6 | P20 | P7 | P21 | P8 | P22 | UART0 | P9 | P23 | GND | P24 | 3V3 | P25 | VIN | P26 | AUX | 5V | P27 | P10 | P28 | P11 | P29 | Ethernet | P12 | P30 | P13 | P31 | HOST
bPlace: 5V | GND | TX2 | RX2 | MPU_RST | REF_CLK | PHY_LED | WLED_N | SCL | SDA | 3V3 | GND | PHY_RDP | RXD1 | PHY_RDN | TXD1 | PHY_TDP | RXD0 | TXD0 | RX1 | TX1 | 3V3 | GND | PHY_TDN | USB_DP | I2C_SDA | USB_DM | I2C_SCL | TXD2 | MOSI | RX0 | TX0 | 3V3 | GND | RXD2 | MISO | SCK | CSI | 3V3 | SPK_VDD | PWM0 | 5V | www.seeedstudio.com | by Seeed Studio | v2.0 03/03/2016 | Breakout for LinkIt Smart 7688 | PWM1 | I2S_WS | MOSI_S | I2S_CLK | MISO_S | I2S_SDI | SCK_S | I2S_SDO | CS_S
bNames: 2:GND / 3:MIC | 2:MIC / 3:GND

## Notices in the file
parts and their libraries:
moudle-new: This work is licensed under the Creative Commons Attribution 4.0 International License.
To view a copy of this license,visit:
http://creativecommons.org/licenses/by-sa/4.0
moudle-new: CC-BY-SA
